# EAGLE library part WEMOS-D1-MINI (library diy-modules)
WEMOS D1 mini: Mini Wi-Fi Board based on ESP-8266 device More details can be found here: https://www.wemos.cc/product/d1-mini.html Click here to find device on ebay.com
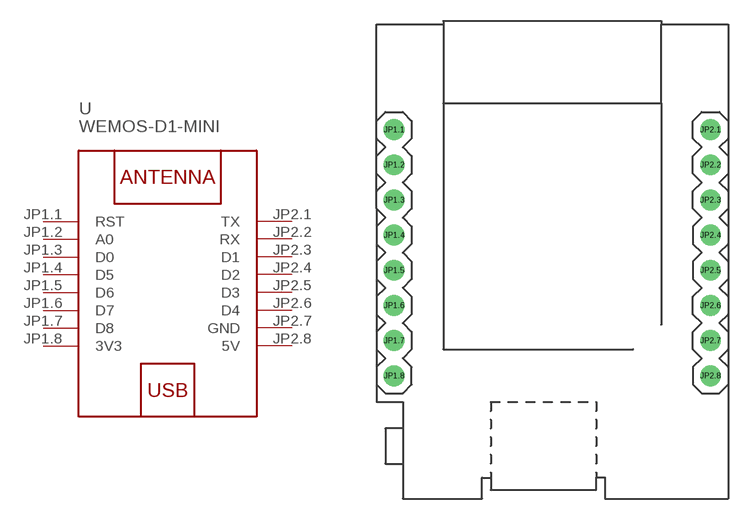
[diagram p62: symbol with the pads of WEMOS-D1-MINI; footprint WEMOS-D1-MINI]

Designator prefix -

## WEMOS-D1-MINI  [WEMOS-D1-MINI]
JP1.1  RST
JP1.2  A0
JP1.3  D0
JP1.4  D5
JP1.5  D6
JP1.6  D7
JP1.7  D8
JP1.8  3V3  pwr
JP2.1  TX
JP2.2  RX
JP2.3  D1
JP2.4  D2
JP2.5  D3
JP2.6  D4
JP2.7  GND  pwr
JP2.8  5V  pwr

## Footprint WEMOS-D1-MINI (pad centres in mm)
WEMOS D1 mini: Mini Wi-Fi Board based on ESP-8266 device
drill 1: JP1.1 -11.43,9.525; JP1.2 -11.43,6.985; JP1.3 -11.43,4.445; JP1.4 -11.43,1.905; JP1.5 -11.43,-0.635; JP1.6 -11.43,-3.175; JP1.7 -11.43,-5.715; JP1.8 -11.43,-8.255; JP2.1 11.43,9.525; JP2.2 11.43,6.985; JP2.3 11.43,4.445; JP2.4 11.43,1.905; JP2.5 11.43,-0.635; JP2.6 11.43,-3.175; JP2.7 11.43,-5.715; JP2.8 11.43,-8.255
